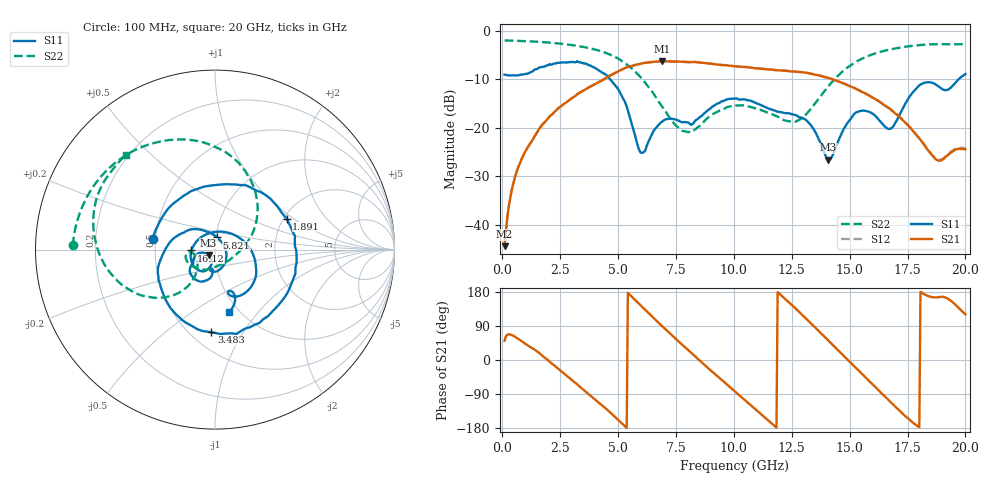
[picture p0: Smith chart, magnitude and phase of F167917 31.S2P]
!  2-Port S-parameters saved by WinCal
! VAR MeasName=S-Parameters (CALIBRATED_DATA) read from VNA (N5242A)
! VAR MeasDate=2016-11-22 9:01:14
! VAR NAME=F167917 31
! VAR FILENAME=F167917 31.S2P
! VAR DATE=2016-11-22 9:01:14
! VAR PHYS_PORTS=1,2
# Hz S DB R 50
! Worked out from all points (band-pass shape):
!   401 points, 100 MHz to 20 GHz, reference 50 ohm
!   highest |S21| = -6.32 dB at 6.916 GHz (marker M1); lowest = -44.4 dB at 100 MHz (marker M2)
!   |S21| within 3 dB of the highest: 4.635 GHz to 13.74 GHz (9.1 GHz wide, 99.1 % of centre)
!   lowest |S11| = -26.6 dB at 14.08 GHz (marker M3), VSWR 1.10, Z = 46.5 - j2.81 ohm
!   |S11| at or under -10 dB: 4.655 GHz to 19.71 GHz (15.06 GHz wide, 124 % of centre)
!   |S22| runs from -20.9 to -2.0 dB; largest |S21 - S12| = 0.0031
!   S11 on the Smith chart (normalised r, x): 100 MHz: 0.48, +0.06; 1.891 GHz: 2.08, +0.89; 3.483 GHz: 0.63, -0.74; 5.821 GHz: 1.01, +0.14; 16.12 GHz: 0.77, -0.01; 20 GHz: 0.90, -0.72
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1e8  -9.07 170.6  -44.44 51.1  -44.40 50.6  -2.02 178.3
6.4725e8  -9.22 124.1  -28.73 57.3  -28.67 57.1  -2.10 169.4
1.891e9  -7.22 23.4  -18.60 3.5  -18.60 3.4  -2.41 148.9
2.488e9  -6.63 -24.4  -15.77 -27.0  -15.77 -26.9  -2.67 138.2
3.43325e9  -6.64 -89.4  -12.57 -74.9  -12.51 -74.8  -3.31 119.4
3.483e9  -6.71 -92.5  -12.44 -77.4  -12.37 -77.3  -3.35 118.3
4.52775e9  -9.27 -158.1  -9.60 -130.8  -9.55 -131.2  -4.70 92.1
5.82125e9  -23.23 80.4  -7.01 153.4  -7.01 153.2  -8.84 49.6
6.07e9  -25.13 22.2  -6.71 138.6  -6.72 138.5  -10.15 40.4
6.7665e9  -19.38 -69.7  -6.34 97.2  -6.35 97.2  -14.74 12.9
6.91575e9  -18.73 -78.4  -6.32 88.4  -6.32 88.4  -15.75 6.7
8.40825e9  -18.33 -96.2  -6.52 4.9  -6.50 4.9  -20.03 -94.1
1.005e10  -14.01 -123.4  -7.34 -83.0  -7.32 -82.9  -15.50 -156.6
1.17415e10  -16.44 -147.8  -8.12 -173.0  -8.08 -173.1  -17.40 -173.4
1.338325e10  -19.90 -166.3  -8.92 93.4  -8.92 93.5  -15.79 -129.8
1.407975e10  -26.60 -139.8  -9.73 51.6  -9.75 51.5  -11.49 -127.1
1.5224e10  -17.06 -119.9  -11.86 -18.0  -11.86 -17.9  -6.59 -146.3
1.61195e10  -17.63 -177.9  -14.13 -71.8  -14.18 -71.6  -4.68 -164.6
1.67165e10  -20.27 105.2  -16.01 -107.8  -16.07 -107.3  -3.91 -176.1
1.776125e10  -12.55 -17.5  -20.85 -166.7  -20.73 -165.6  -3.10 165.8
1.875625e10  -11.22 -70.4  -26.66 165.2  -26.47 166.0  -2.80 149.7
2e10  -8.95 -77.5  -24.43 120.4  -24.22 120.6  -2.79 133.4
